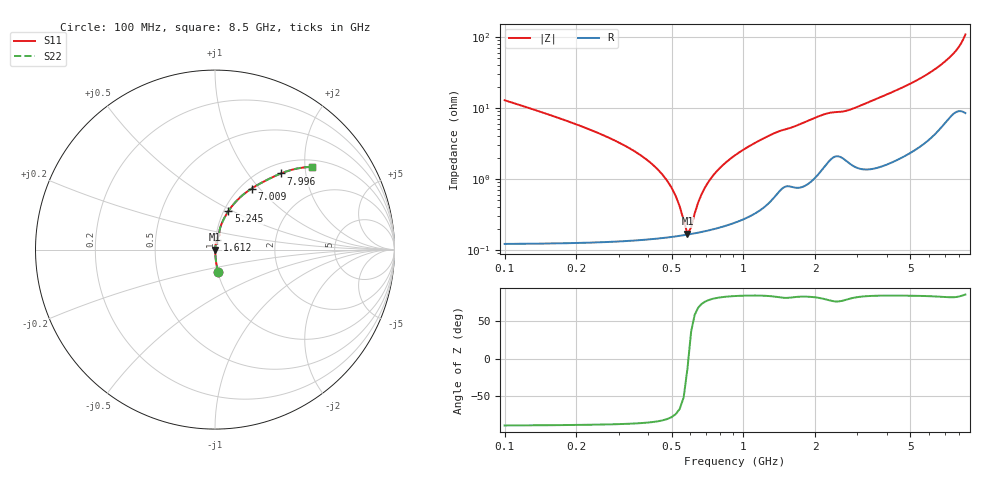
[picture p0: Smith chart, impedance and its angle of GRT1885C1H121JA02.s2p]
!Murata Part Number: GRT1885C1H121JA02
!These Parameters are Measured in Series Mode Connection
!Data Generated on Jun 19, 2026
!  o--ll--o
!Port1  Port2
!  o------o
!Operation Temp=25[degC], DC Bias Voltage=0[V]
!Freq. Start=100[MHz] Stop=9[GHz] 401[Steps]
# Hz S RI R 50
!Freq.(Hz) S11(Real) S11(Imag) S21(Real) S21(Imag) S12(Real) S12(Imag) S22(Real) S22(Imag)
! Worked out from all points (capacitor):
!   401 points, 100 MHz to 8.5 GHz, reference 50 ohm
!   read as one part in series: C = 120 pF near 142 MHz
!   lowest |Z| = 169 mohm at 583 MHz (marker M1)
!   series resonance near 588.1 MHz, so ESL is about 610 pH
!   S11 on the Smith chart (normalised r, x): 100 MHz: 1.00, -0.26; 1.612 GHz: 1.02, +0.11; 5.245 GHz: 1.05, +0.48; 7.009 GHz: 1.12, +0.91; 7.996 GHz: 1.18, +1.46; 8.5 GHz: 1.17, +2.17
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1e8  0.0175 -0.1264  0.9825 0.1264  0.9825 0.1264  0.0175 -0.1264
4.36e8  0.00163 -0.0137  0.9984 0.0137  0.9984 0.0137  0.00163 -0.0137
4.99e8  0.00157 -0.00745  0.9984 0.00745  0.9984 0.00745  0.00157 -0.00745
5.62e8  0.00161 -0.00205  0.9984 0.00205  0.9984 0.00205  0.00161 -0.00205
5.83e8  0.00164 -0.000388  0.9984 0.000388  0.9984 0.000388  0.00164 -0.000388
6.04e8  0.00167 0.00122  0.9983 -0.00122  0.9983 -0.00122  0.00167 0.00122
6.25e8  0.00171 0.00277  0.9983 -0.00277  0.9983 -0.00277  0.00171 0.00277
6.67e8  0.00182 0.00574  0.9982 -0.00574  0.9982 -0.00574  0.00182 0.00574
7.3e8  0.00201 0.00991  0.998 -0.00991  0.998 -0.00991  0.00201 0.00991
8.56e8  0.00252 0.0176  0.9975 -0.0176  0.9975 -0.0176  0.00252 0.0176
1.129e9  0.00436 0.0324  0.9956 -0.0324  0.9956 -0.0324  0.00436 0.0324
1.507e9  0.0102 0.0488  0.9898 -0.0488  0.9898 -0.0488  0.0102 0.0488
1.612e9  0.0104 0.0525  0.9896 -0.0525  0.9896 -0.0525  0.0104 0.0525
2.179e9  0.0206 0.0775  0.9794 -0.0775  0.9794 -0.0775  0.0206 0.0775
2.914e9  0.024 0.0949  0.976 -0.0949  0.976 -0.0949  0.024 0.0949
4.3e9  0.0451 0.1622  0.9549 -0.1622  0.9549 -0.1622  0.0451 0.1622
5.245e9  0.0751 0.2151  0.9249 -0.2151  0.9249 -0.2151  0.0751 0.2151
5.707e9  0.0967 0.2447  0.9033 -0.2447  0.9033 -0.2447  0.0967 0.2447
7.009e9  0.2042 0.3403  0.7958 -0.3403  0.7958 -0.3403  0.2042 0.3403
7.114e9  0.2171 0.3484  0.7829 -0.3484  0.7829 -0.3484  0.2171 0.3484
7.996e9  0.3671 0.4241  0.6329 -0.4241  0.6329 -0.4241  0.3671 0.4241
8.5e9  0.5398 0.4609  0.4602 -0.4609  0.4602 -0.4609  0.5398 0.4609
